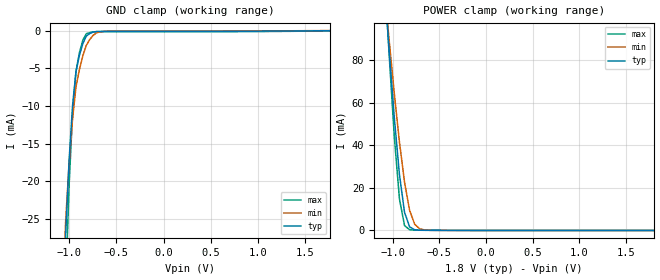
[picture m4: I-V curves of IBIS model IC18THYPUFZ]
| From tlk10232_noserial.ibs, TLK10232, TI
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[Model]   IC18THYPUFZ
Model_type   Input
Polarity   Non-Inverting
Vinl =  0.63
Vinh =  1.17
C_comp   0.6359007p   0.5293641p   0.7739418p
[Model Spec]
Vinl   0.63   0.567   0.693
Vinh   1.17   1.053   1.287
[Temperature Range]   25   125   -40
[Voltage Range]   1.8   1.62   1.98
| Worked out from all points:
|   GND clamp passes 1 mA (typ) near -0.83 V on its own axis
|   POWER clamp passes 1 mA (typ) near -0.79 V on its own axis
[POWER_clamp]
-1.8V     607.5mA    493.2mA    734.2mA
-1.055V   94.9mA     97.36mA    95.3mA
-1.036V   83.71mA    88.66mA    81.38mA
-981.8mV  52.63mA    63.94mA    43.63mA
-927.3mV  26.21mA    41.44mA    14.78mA
-872.7mV  8.503mA    22.57mA    2.281mA
-818.2mV  1.687mA    9.395mA    320.8uA
-763.6mV  321.1uA    2.894mA    143.8uA
-709.1mV  115.9uA    758.6uA    121.8uA
-654.5mV  82.76uA    210.9uA    111.2uA
1.8V      92.69pA    83.97pA    102.7pA
[GND_clamp]
-1.8V     -542mA     -381.7mA   -757.7mA
-1.073V   -42.85mA   -36.01mA   -57.34mA
-1.036V   -26.91mA   -25.11mA   -33.87mA
-1V       -17.09mA   -17.59mA   -20.42mA
-963.6mV  -9.93mA    -11.69mA   -10.92mA
-927.3mV  -5.413mA   -7.429mA   -5.37mA
-890.9mV  -3.269mA   -5.135mA   -2.902mA
-854.5mV  -1.703mA   -3.308mA   -1.248mA
-818.2mV  -714uA     -1.949mA   -411uA
-709.1mV  -111.3uA   -277.2uA   -149.7uA
-600mV    -90.19uA   -59.14uA   -147.9uA
1.764V    -3.961uA   10.1uA     -32.99uA
